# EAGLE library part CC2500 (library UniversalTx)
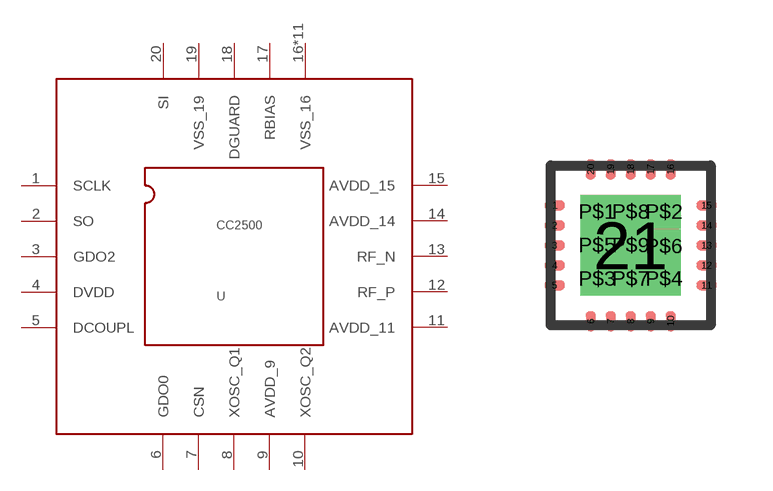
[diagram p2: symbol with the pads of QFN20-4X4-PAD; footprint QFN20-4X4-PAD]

Designator prefix -

## CC2500  [QFN20-4X4-PAD]
1  SCLK
2  SO
3  GDO2
4  DVDD
5  DCOUPL
6  GDO0
7  CSN
8  XOSC_Q1
9  AVDD_9
10  XOSC_Q2
11  AVDD_11
12  RF_P
13  RF_N
14  AVDD_14
15  AVDD_15
16  VSS_16
17  RBIAS
18  DGUARD
19  VSS_19
20  SI
21  VSS_16
P$1  VSS_16
P$2  VSS_16
P$3  VSS_16
P$4  VSS_16
P$5  VSS_16
P$6  VSS_16
P$7  VSS_16
P$8  VSS_16
P$9  VSS_16

## Footprint QFN20-4X4-PAD (pad centres in mm)
QFN20 4mm x 4mm package, with matt tin plating from Nordic Semiconductor.
smd 0.5 x 0.25: 1 -1.9,1; 2 -1.9,0.5; 3 -1.9,0; 4 -1.9,-0.5; 5 -1.9,-1; 11 1.9,-1; 12 1.9,-0.5; 13 1.9,0; 14 1.9,0.5; 15 1.9,1
smd 0.25 x 0.5: 6 -1,-1.9; 7 -0.5,-1.9; 8 0,-1.9; 9 0.5,-1.9; 10 1,-1.9; 16 1,1.9; 17 0.5,1.9; 18 0,1.9; 19 -0.5,1.9; 20 -1,1.9
smd 2.4 x 2.4: 21 0,0
drill 0.33 pad 0.686 square: P$1 -0.838,0.838; P$2 0.838,0.838; P$3 -0.838,-0.838; P$4 0.838,-0.838; P$5 -0.838,0; P$6 0.838,-0.025; P$7 0,-0.838; P$8 0,0.838; P$9 0,0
